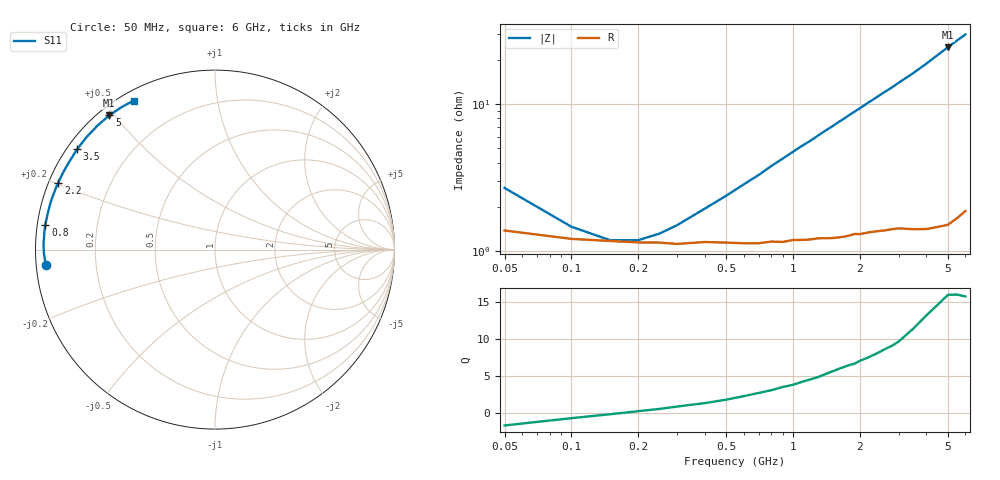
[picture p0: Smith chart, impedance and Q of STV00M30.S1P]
! SIEMENS Discrete & RF Semiconductors
! BA892
! Si PIN Diode in SCD-80
! IF = 0.3 mA
! S-Parameters:  September  1997
# GHz  S  MA  R  50
!  f  S11
! GHz  MAG  ANG
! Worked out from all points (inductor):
!   34 points, 50 MHz to 6 GHz, reference 50 ohm
!   read as one part to ground: L = 731 pH near 800 MHz
!   highest Q = 16 at 5 GHz (marker M1), where L = 772 pH
!   S11 on the Smith chart (normalised r, x): 50 MHz: 0.03, -0.05; 800 MHz: 0.02, +0.07; 2.2 GHz: 0.03, +0.20; 3.5 GHz: 0.03, +0.32; 5 GHz: 0.03, +0.49; 6 GHz: 0.04, +0.59
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0.05  0.9461 -174.7
0.1  0.9525 -178.1
0.15  0.954 -179.6
0.2  0.955 179.3
0.3  0.956 177.7
0.4  0.9547 176.4
0.6  0.9557 174.0
0.7  0.9557 172.9
0.8  0.9546 171.7
0.9  0.9549 170.6
1.1  0.9537 168.4
1.2  0.9535 167.4
1.4  0.9528 165.2
1.5  0.9528 164.2
1.6  0.9525 163.1
1.8  0.9513 161.0
2  0.9506 159.0
2.2  0.9496 156.9
2.4  0.9491 154.9
2.6  0.9488 152.9
2.8  0.9483 151.0
3  0.9481 148.9
3.5  0.9501 144.0
4  0.9515 138.8
4.5  0.9517 133.4
5  0.9521 128.2
5.5  0.9492 123.2
6  0.9459 118.6
